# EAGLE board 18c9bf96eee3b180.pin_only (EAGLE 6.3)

Size 35.56 x 29.21 mm. Coordinates in mm from the lower left corner, seen from the top.
Outline: 0,26.67 0,2.54 arc90 2.54,0 33.02,0 arc90 35.56,2.54 35.56,26.67 arc90 33.02,29.21 2.54,29.21 arc90 0,26.67
Copper layers (1*16): Top 0.035mm / dielectric 1.5mm / Bottom 0.035mm
Design rules "pcbcart *": minimum track width 8mil, minimum drill 0.4mm, track to track 10mil, track to pad 10mil, pad to pad 10mil, via to via 10mil, smd to smd 8mil, copper to edge 20mil, drill to drill 8mil, minimum pad ring 8mil, minimum via ring 10mil, stop-mask expansion 3mil, vias tented up to drill 25mil, thermal gap 8mil

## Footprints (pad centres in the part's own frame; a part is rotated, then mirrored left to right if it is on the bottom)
0805 = smd 1.3 x 1.5: 1 -0.95,0; 2 0.95,0
MICROSD = smd 0.7 x 1.5: 1 9,-10.64; 2 7.9,-10.24; 3 6.8,-10.64; 4 5.7,-11.04; 5 4.6,-10.64; 6 3.5,-11.04; 7 2.4,-10.64; 8 1.3,-10.64 | smd 1.8 x 1.4: CD1 2,-0.44; CD2 8,-0.44 | smd 1.4 x 1.9: MT1 0.4,-13.54; MT2 13.6,-14.44
SOD-123 = smd 1.4 x 1.4: A 1.85,0; C -1.85,0
SOT23-5L = smd 0.55 x 1.2: 1 -0.95,-1.3; 2 0,-1.3; 3 0.95,-1.3; 4 0.95,1.3; 5 -0.95,1.3
1X10_ROUND_76 = drill 1 pad 1.93 square: 1 -11.43,0 | drill 1 pad 1.93: 2 -8.89,0; 3 -6.35,0; 4 -3.81,0; 5 -1.27,0; 6 1.27,0; 7 3.81,0; 8 6.35,0; 9 8.89,0; 10 11.43,0
INDUCTOR_1007 = smd 1.016 x 2.2: P$1 -1.127,0; P$2 1.127,0
UG-9664HDDAG01_WRAPAROUND = smd 0.35 x 3 bottom: 1 -7.7,4.138; 2 -7,4.138; 3 -6.3,4.138; 4 -5.6,4.138; 5 -4.9,4.138; 6 -4.2,4.138; 7 -3.5,4.138; 8 -2.8,4.138; 9 -2.1,4.138; 10 -1.4,4.138; 11 -0.7,4.138; 12 0,4.138; 13 0.7,4.138; 14 1.4,4.138; 15 2.1,4.138; 16 2.8,4.138; 17 3.5,4.138; 18 4.2,4.138; 19 4.9,4.138; 20 5.6,4.138; 21 6.3,4.138; 22 7,4.138; 23 7.7,4.138 | hole 1: -8,0.688; 8,0.688
SOT23-5 = smd 0.55 x 1.2: 1 -0.95,-1.3; 2 0,-1.3; 3 0.95,-1.3; 4 0.95,1.3; 5 -0.95,1.3
SOIC16 = smd 0.6 x 2.2: 1 -4.445,-2.6; 2 -3.175,-2.6; 3 -1.905,-2.6; 4 -0.635,-2.6; 5 0.635,-2.6; 6 1.905,-2.6; 7 3.175,-2.6; 8 4.445,-2.6; 9 4.445,2.6; 10 3.175,2.6; 11 1.905,2.6; 12 0.635,2.6; 13 -0.635,2.6; 14 -1.905,2.6; 15 -3.175,2.6; 16 -4.445,2.6
MOUNTINGHOLE_2.5_PLATED = drill 2.5 pad 3.2: P$1 0,0
FIDUCIAL_1MM = smd 1 x 1: 1 0,0

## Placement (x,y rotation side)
C1  10uF  [0805]  33.39,18.29 90 top
C2  0.1uF  [0805]  32.26,8.52 0 top
C3  10uF/16V  [0805]  7.87,6.73 90 top
C4  10uF/16V  [0805]  28.96,3.68 270 top
C5  10uF/16V  [0805]  5.58,6.73 90 top
C8  10uF  [0805]  29.46,16.76 0 top
CN1  [MICROSD]  16.13,23.5 270 top
D1  BAT54T1G  [SOD-123]  28.82,9.65 90 top
IC1  MIC5225-3.3  [SOT23-5L]  29.46,19.56 90 top
JP2  [1X10_ROUND_76]  17.73,26.75 180 bottom
L1  10uH  [INDUCTOR_1007]  29.45,14.02 180 top
LCD1  UG-9664HDDAG01  [UG-9664HDDAG01_WRAPAROUND]  17.78,1.81 0 bottom
R1  100K  [0805]  32.26,10.66 180 top
R2  10K  [0805]  32.26,6.36 0 top
R3  920K  [0805]  19.69,11.18 270 top
U1  FAN5331SX  [SOT23-5]  33.02,14.11 0 top
U2  74HC4050  [SOIC16]  22.1,17.4 180 top
U$9  MOUNTINGHOLE2.5  [MOUNTINGHOLE_2.5_PLATED]  2.54,26.67 0 bottom
U$10  MOUNTINGHOLE2.5  [MOUNTINGHOLE_2.5_PLATED]  2.54,2.54 0 top
U$11  MOUNTINGHOLE2.5  [MOUNTINGHOLE_2.5_PLATED]  33.02,26.67 0 bottom
U$12  FIDUCIAL  [FIDUCIAL_1MM]  5.33,1.28 0 top
U$13  FIDUCIAL  [FIDUCIAL_1MM]  1.78,20.71 0 top
U$15  MOUNTINGHOLE2.5  [MOUNTINGHOLE_2.5_PLATED]  33.02,2.54 0 top
U$16  FIDUCIAL  [FIDUCIAL_1MM]  34.16,23.5 0 top
U$17  [ADAFRUIT_3.5MM]  0.51,5.08 0 top
U$28  [LOGIC_5VREADY_5MM]  21.21,8.13 0 top

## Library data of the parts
C1-C5 C8 CN1 D1 JP2 L1 LCD1 R1-R3 U1 U2 U$9-U$11 U$15 U$17 U$28 = microbuilder
IC1 U$12 U$13 U$16 = adafruit

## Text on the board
tPlace: MISO | SCK | RST | SDCS | GND | CD | MOSI | D/C | OCS | VCC | from adafruit!
bPlace: SSD1331 96x64 SPI RGB OLED | CD | SO | SI | CK | DC | R | OC | SC | + | G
